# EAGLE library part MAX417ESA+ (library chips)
Maxim Dual Single Supply Op Amp
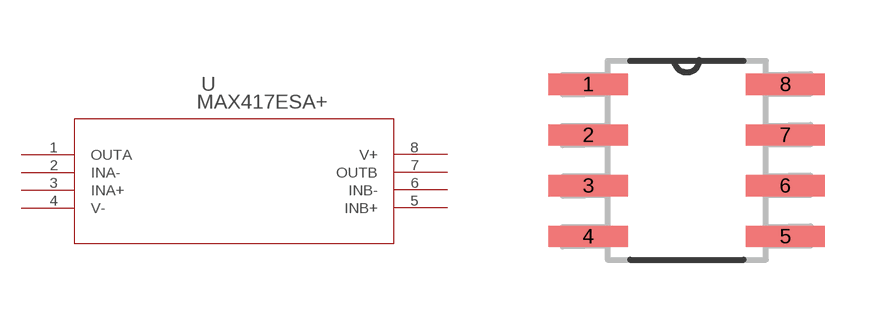
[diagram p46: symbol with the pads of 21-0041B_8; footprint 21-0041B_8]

Designator prefix U

## MAX417ESA+ (MANUFACTURER: MAXIM; MPN: max417esa+)  [21-0041B_8]
1  OUTA  out
2  INA-  in
3  INA+  in
4  V-  pwr
5  INB+  in
6  INB-  in
7  OUTB  out
8  V+  pwr

## Footprint 21-0041B_8 (pad centres in mm)
smd 1.981 x 0.533: 1 -2.464,1.905; 2 -2.464,0.635; 3 -2.464,-0.635; 4 -2.464,-1.905; 5 2.464,-1.905; 6 2.464,-0.635; 7 2.464,0.635; 8 2.464,1.905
